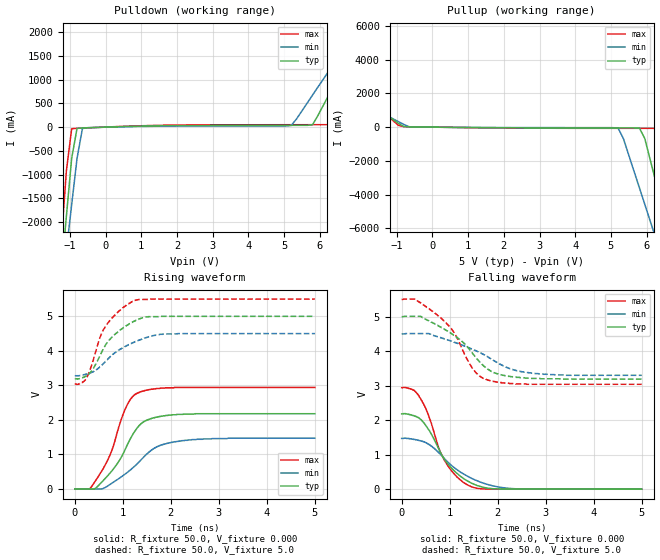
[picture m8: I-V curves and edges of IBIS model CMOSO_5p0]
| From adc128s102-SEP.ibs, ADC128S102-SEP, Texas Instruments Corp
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|   Model CMOSO_5p0
[Model]  CMOSO_5p0
Model_type Output
Enable   Active-High
Vmeas =  1
C_comp   73.44fF   64.02fF   74.18fF
[Temperature Range]   25.000   105.000   -40.000
[Voltage Range]   5.0V   4.50V   5.50V
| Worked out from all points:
|   slope of the pulldown table from 0 to 0.75 V, typ, clamps not added: 43.8 ohm
|   slope of the pullup table from 0 to 0.75 V, typ, clamps not added: 43.6 ohm
|   rising waveform, R_fixture 50.0, V_fixture 0.000: 20-80 % time 568ps typ, 739ps min, 473ps max; typ from 0 V to 2.18 V
|   rising waveform, R_fixture 50.0, V_fixture 5.0: 20-80 % time 568ps typ, 726ps min, 476ps max; typ from 3.19 V to 5 V
|   falling waveform, R_fixture 50.0, V_fixture 0.000: 20-80 % time 615ps typ, 803ps min, 510ps max; typ from 2.18 V to 0 V
|   falling waveform, R_fixture 50.0, V_fixture 5.0: 20-80 % time 833ps typ, 1.09ns min, 683ps max; typ from 5 V to 3.19 V
[Pulldown]
|Voltage   I(typ)   I(min)   I(max)
-5V       -34A       -28A       -42A
-1.25V    -3.13A     -3.58A     -2.51A
-1.1V     -1.89A     -2.61A     -931mA
-950mV    -654mA     -1.63A     -33.3mA
-800mV    -25.8mA    -656mA     -25.3mA
-650mV    -17.3mA    -30.2mA    -20.5mA
5.2V      37.1mA     35.5mA     50.7mA
5.8V      52mA       677mA      51.2mA
6.25V     673mA      1.18A      52.2mA
7V        1.74A      2.03A      1.23A
7.45V     2.39A      2.53A      2.05A
10V       6.04A      5.42A      6.7A
[Pullup]
|Voltage   I(typ)   I(min)   I(max)
-5V       5.97A      4.87A      7.42A
-4.1V     4.69A      3.85A      5.8A
-950mV    223mA      322mA      105mA
-500mV    13.2mA     9.82mA     17.4mA
5.2V      -49.2mA    -51.9mA    -71.1mA
5.8V      -57mA      -3.61A     -71.9mA
5.95V     -689mA     -4.59A     -72.1mA
6.1V      -1.93A     -5.57A     -72.2mA
6.4V      -4.41A     -7.52A     -78.7mA
6.55V     -5.65A     -8.5A      -980mA
7V        -9.37A     -11.4A     -5.74A
10V       -34.1A     -30.9A     -37.4A
[Ramp]
|variable   typ   min   max
dV/dt_r   1.309V/568.5p   883.8mV/744.6p   1.766V/473.9p
dV/dt_f   1.310V/614.5p   883.9mV/804.3p   1.766V/510.9p
R_load  = 50
[Rising Waveform]
R_fixture = 50.0
V_fixture = 0.000
V_fixture_min = 0.000
V_fixture_max = 0.000
|  time   V(typ)   V(min)   V(max)
0s        89.3pV     5.92nV     81.5pV
300ps     -1.64mV    -2.59mV    2.04mV
480ps     80.2mV     -1.82mV    339mV
745ps     478mV      142mV      1.02V
935ps     840mV      319mV      1.88V
1.085ns   1.25V      470mV      2.42V
1.32ns    1.8V       757mV      2.79V
1.715ns   2.08V      1.23V      2.91V
2.17ns    2.16V      1.39V      2.94V
5ns       2.18V      1.47V      2.94V
[Rising Waveform]
R_fixture = 50.0
V_fixture = 5.0
V_fixture_min = 4.5
V_fixture_max = 5.5
|  time   V(typ)   V(min)   V(max)
0s        3.19V      3.28V      3.04V
150ps     3.22V      3.3V       3.08V
255ps     3.28V      3.33V      3.24V
395ps     3.51V      3.41V      3.78V
530ps     3.88V      3.54V      4.41V
695ps     4.27V      3.77V      4.82V
1.01ns    4.67V      4.1V       5.26V
1.265ns   4.88V      4.27V      5.47V
1.845ns   5V         4.49V      5.5V
5ns       5V         4.5V       5.5V
[Falling Waveform]
R_fixture = 50.0
V_fixture = 0.000
V_fixture_min = 0.000
V_fixture_max = 0.000
|  time   V(typ)   V(min)   V(max)
0s        2.18V      1.47V      2.94V
325ps     2.09V      1.42V      2.77V
530ps     1.79V      1.33V      2.25V
795ps     1.1V       1.03V      1.11V
885ps     877mV      896mV      852mV
1.135ns   477mV      580mV      376mV
1.43ns    190mV      331mV      84.3mV
1.79ns    29.7mV     136mV      3.45mV
2.29ns    1.83mV     17.8mV     799uV
5ns       135uV      266uV      78.7uV
[Falling Waveform]
R_fixture = 50.0
V_fixture = 5.0
V_fixture_min = 4.5
V_fixture_max = 5.5
|  time   V(typ)   V(min)   V(max)
0s        5V         4.5V       5.5V
295ps     5.01V      4.51V      5.51V
570ps     4.88V      4.51V      5.23V
860ps     4.66V      4.37V      4.91V
1.11ns    4.44V      4.25V      4.5V
1.495ns   3.9V       4.04V      3.46V
1.795ns   3.48V      3.83V      3.16V
2.215ns   3.28V      3.51V      3.07V
2.705ns   3.21V      3.36V      3.04V
5ns       3.19V      3.3V       3.04V
